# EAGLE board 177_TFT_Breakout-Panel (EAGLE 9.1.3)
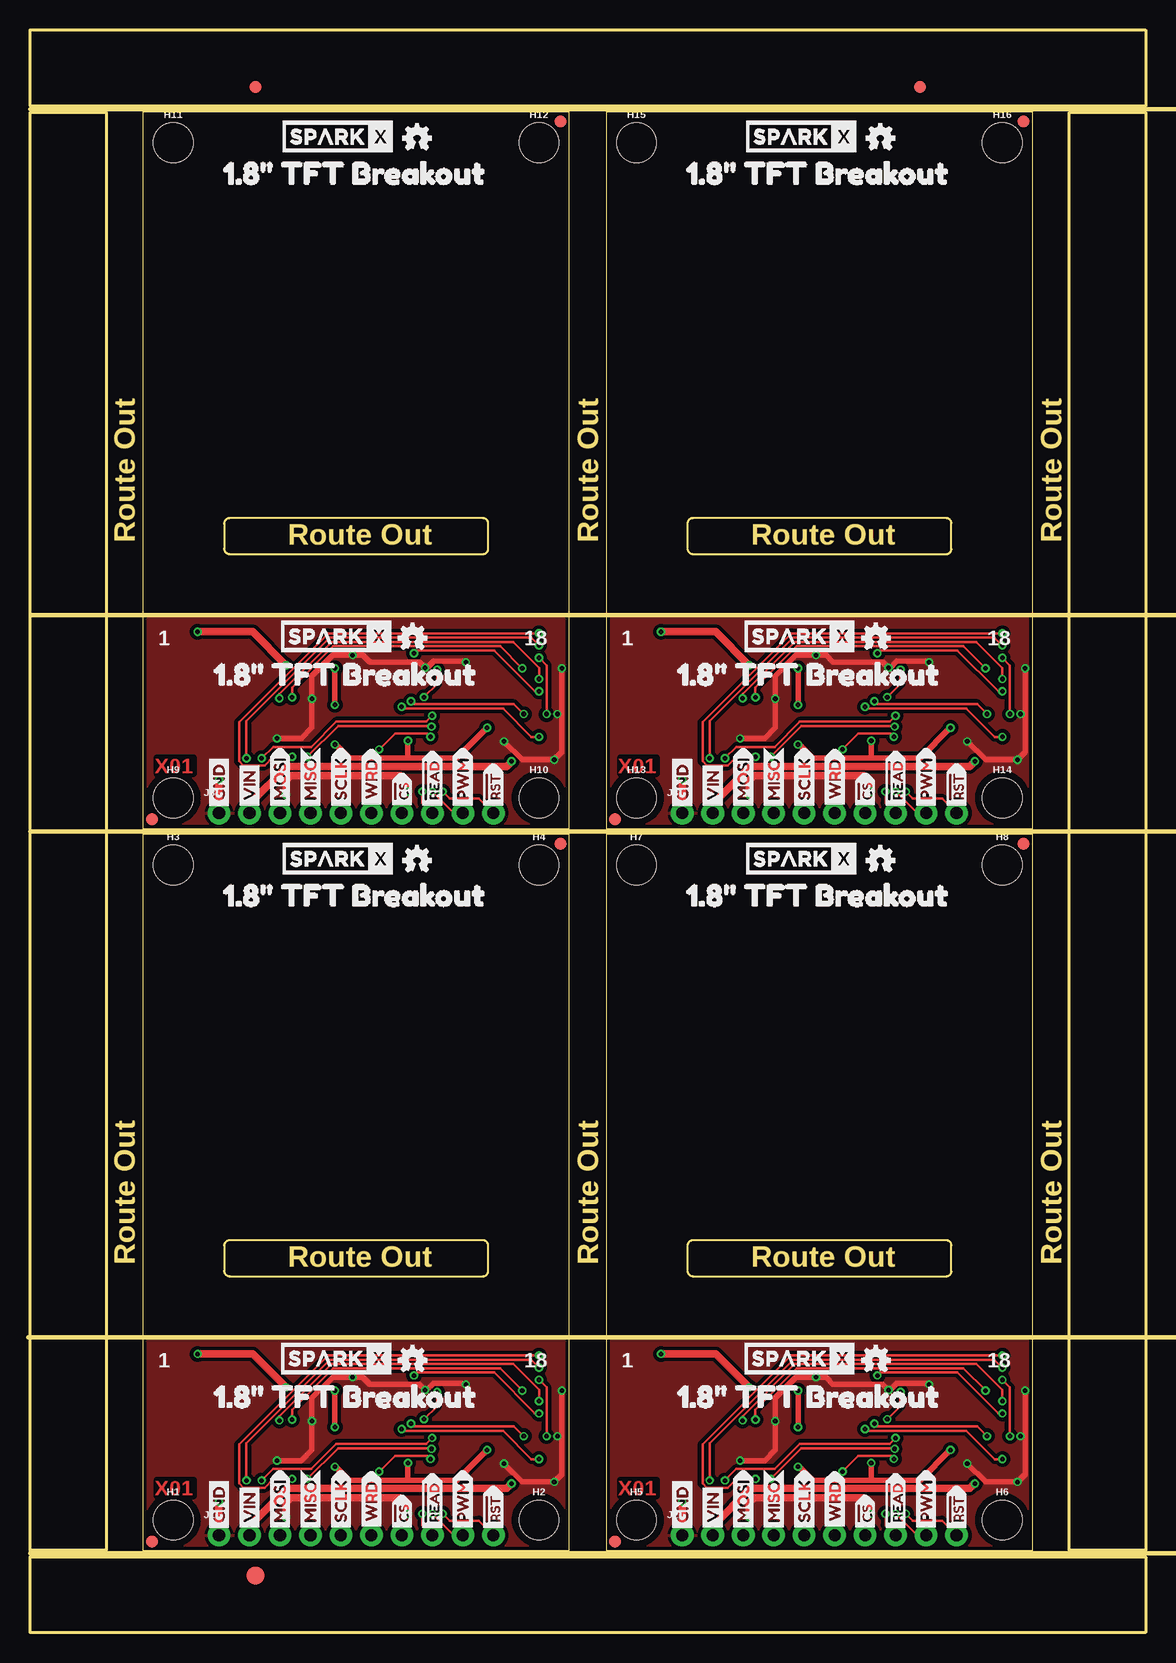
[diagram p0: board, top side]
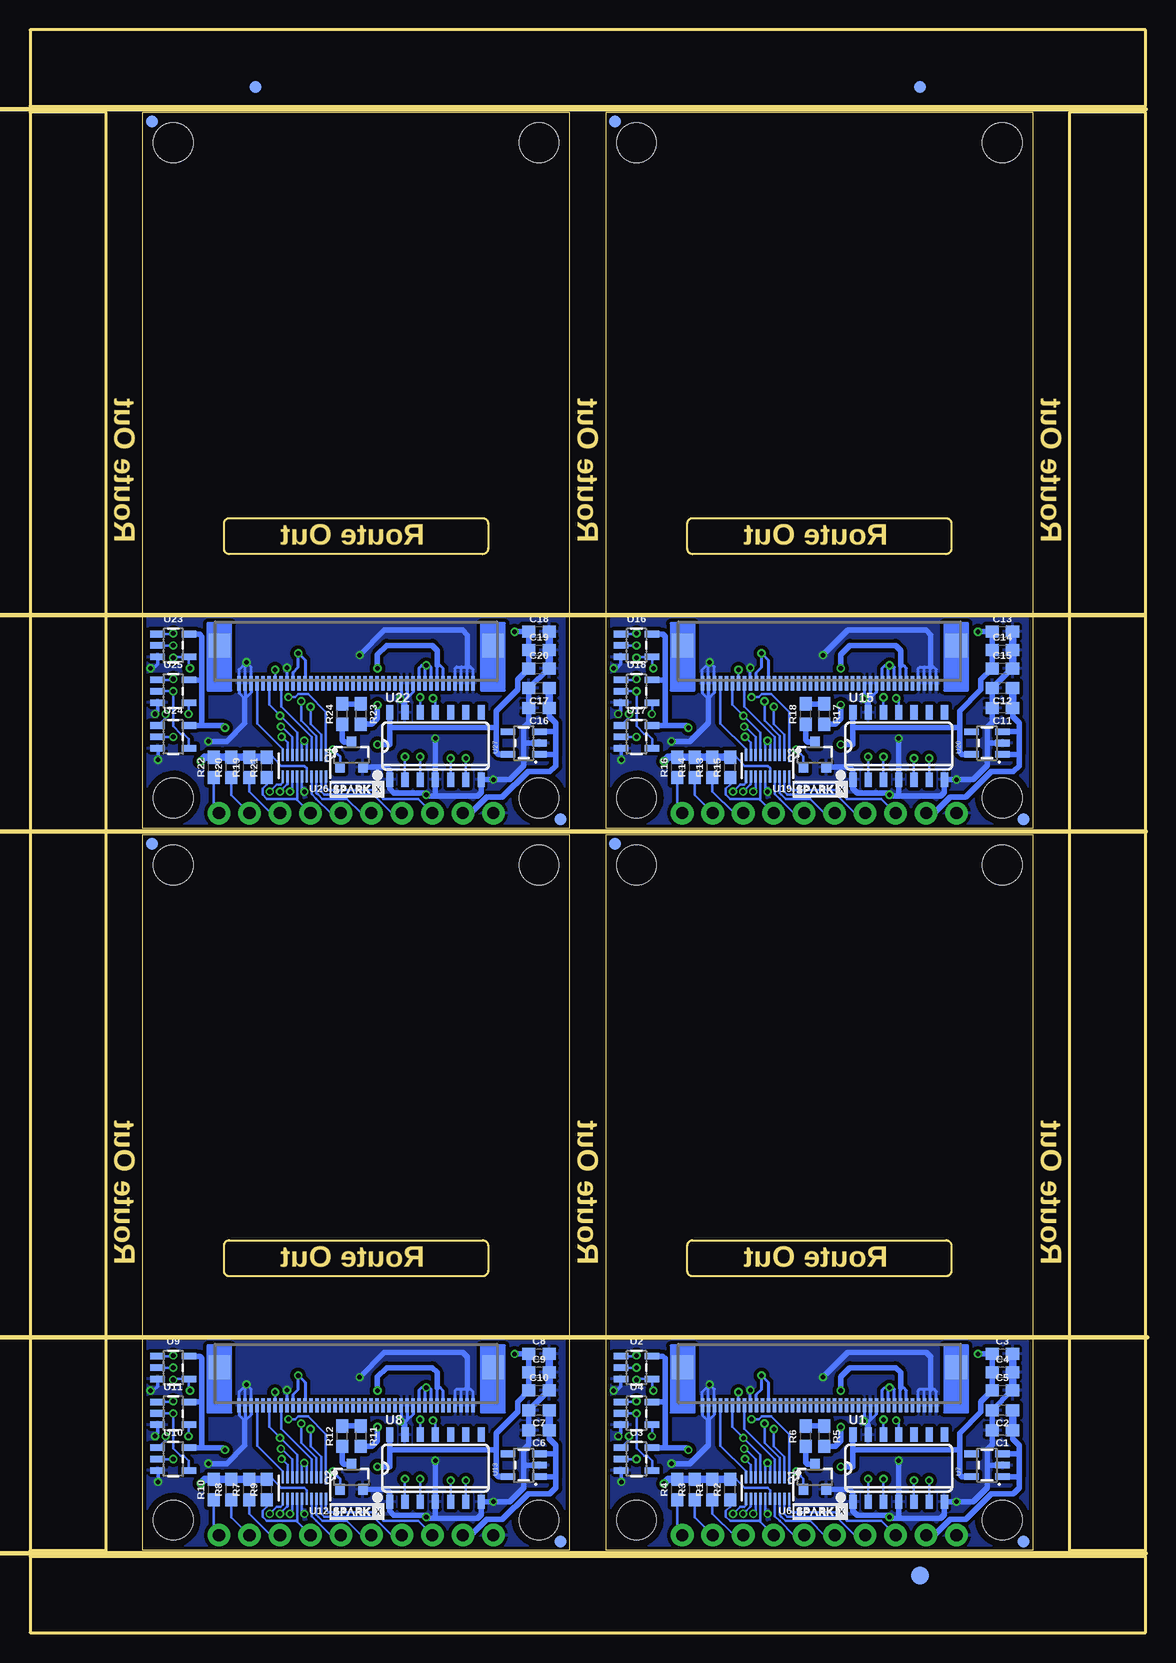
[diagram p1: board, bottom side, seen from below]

Size 92.96 x 133.6 mm. Coordinates in mm from the lower left corner, seen from the top.
Outline: 9.4,6.86 44.96,6.86 44.96,66.55 9.4,66.55 9.4,6.86
Outline: 48.01,6.86 83.57,6.86 83.57,66.55 48.01,66.55 48.01,6.86
Outline: 9.4,67.06 44.96,67.06 44.96,126.75 9.4,126.75 9.4,67.06
Outline: 48.01,67.06 83.57,67.06 83.57,126.75 48.01,126.75 48.01,67.06
Outline: 0,6.35 92.96,6.35 92.96,0 0,0 0,6.35
Outline: 86.61,126.75 92.96,126.75 92.96,6.86 86.61,6.86 86.61,126.75
Outline: 0,133.6 92.96,133.6 92.96,127.25 0,127.25 0,133.6
Outline: 0,126.75 6.35,126.75 6.35,6.86 0,6.86 0,126.75
Copper layers (1*16): Top 0.035mm / dielectric 1.5mm / Bottom 0.035mm
Design rules "SparkFun-2-layer-PCBWay-LIMIT": minimum track width 6mil, minimum drill 0.3mm, track to track 6mil, track to pad 6mil, pad to pad 6mil, via to via 6mil, smd to smd 6mil, copper to edge 6mil, drill to drill 6mil, minimum pad ring 6mil, minimum via ring 6mil, stop-mask expansion 4mil, vias tented up to drill 25mil, thermal gap 10mil
Milling: 37 lines

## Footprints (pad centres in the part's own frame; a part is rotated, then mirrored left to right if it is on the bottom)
0603 = smd 1.1 x 1: 1 -0.85,0; 2 0.85,0
FIDUCIAL-1X2 = smd 1 x 1: 1 0,0
FIDUCIAL-1.5X3 = smd 1.5 x 1.5: 1 0,0
STAND-OFF = hole 3.302: 0,0
1X10_NO_SILK = drill 1.016 pad 1.88: 1 0,0; 2 2.54,0; 3 5.08,0; 4 7.62,0; 5 10.16,0; 6 12.7,0; 7 15.24,0; 8 17.78,0; 9 20.32,0; 10 22.86,0
SOT23-3 = smd 0.8 x 0.9: 1 -0.95,-1; 2 0.95,-1; 3 0,1.1
SO14 = smd 0.6 x 1.2: 1 -3.175,-2.8; 2 -1.905,-2.8; 3 -0.635,-2.8; 4 0.635,-2.8; 5 1.905,-2.8; 6 3.175,-2.8; 7 4.445,-2.8; 8 4.445,2.8; 9 3.175,2.8; 10 1.905,2.8; 11 0.635,2.8; 12 -0.635,2.8; 13 -1.905,2.8; 14 -3.175,2.8
SOT23-5 = smd 0.55 x 1.2: 1 -0.95,-1.3; 2 0,-1.3; 3 0.95,-1.3; 4 0.95,1.3; 5 -0.95,1.3
FPC05040-17204 = smd 0.3 x 1.2: P$1 -9.75,0.6; P$2 -9.25,0.6; P$3 -8.75,0.6; P$4 -8.25,0.6; P$5 -7.75,0.6; P$6 -7.25,0.6; P$7 -6.75,0.6; P$8 -6.25,0.6; P$9 -5.75,0.6; P$10 -5.25,0.6; P$11 -4.75,0.6; P$12 -4.25,0.6; P$13 -3.75,0.6; P$14 -3.25,0.6; P$15 -2.75,0.6; P$16 -2.25,0.6; P$17 -1.75,0.6; P$18 -1.25,0.6; P$19 -0.75,0.6; P$20 -0.25,0.6; P$21 0.25,0.6; P$22 0.75,0.6; P$23 1.25,0.6; P$24 1.75,0.6; P$25 2.25,0.6; P$26 2.75,0.6; P$27 3.25,0.6; P$28 3.75,0.6; P$29 4.25,0.6; P$30 4.75,0.6; P$31 5.25,0.6; P$32 5.75,0.6; P$33 6.25,0.6; P$34 6.75,0.6; P$35 7.25,0.6; P$36 7.75,0.6; P$37 8.25,0.6; P$38 8.75,0.6; P$39 9.25,0.6; P$40 9.75,0.6 | smd 1.8 x 2: P$41 -11.4,-2.55; P$42 11.4,-2.55
UFDFN-20 = smd 0.2 x 1.1: 1 -1.8,-0.85 | smd 0.2 x 1: 2 -1.4,-0.9; 3 -1,-0.9; 4 -0.6,-0.9; 5 -0.2,-0.9; 6 0.2,-0.9; 7 0.6,-0.9; 8 1,-0.9; 9 1.4,-0.9; 10 1.8,-0.9; 11 1.8,0.9; 12 1.4,0.9; 13 1,0.9; 14 0.6,0.9; 15 0.2,0.9; 16 -0.2,0.9; 17 -0.6,0.9; 18 -1,0.9; 19 -1.4,0.9; 20 -1.8,0.9

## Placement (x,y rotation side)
C1  0.1uF  [0603]  11.94,16.89 180 bottom
C2  1.0uF  [0603]  11.94,18.54 180 bottom
C3  4.7uF  [0603]  11.94,23.24 0 bottom
C4  1.0uF  [0603]  11.94,21.72 0 bottom
C5  0.1uF  [0603]  11.94,20.19 0 bottom
C6  0.1uF  [0603]  50.55,16.89 180 bottom
C7  1.0uF  [0603]  50.55,18.54 180 bottom
C8  4.7uF  [0603]  50.55,23.24 0 bottom
C9  1.0uF  [0603]  50.55,21.72 0 bottom
C10  0.1uF  [0603]  50.55,20.19 0 bottom
C11  0.1uF  [0603]  11.94,77.09 180 bottom
C12  1.0uF  [0603]  11.94,78.74 180 bottom
C13  4.7uF  [0603]  11.94,83.44 0 bottom
C14  1.0uF  [0603]  11.94,81.92 0 bottom
C15  0.1uF  [0603]  11.94,80.39 0 bottom
C16  0.1uF  [0603]  50.55,77.09 180 bottom
C17  1.0uF  [0603]  50.55,78.74 180 bottom
C18  4.7uF  [0603]  50.55,83.44 0 bottom
C19  1.0uF  [0603]  50.55,81.92 0 bottom
C20  0.1uF  [0603]  50.55,80.39 0 bottom
E$1  [FIDUCIAL-1X2]  18.8,128.84 0 top
E$2  [FIDUCIAL-1X2]  18.8,128.84 0 bottom
E$3  [FIDUCIAL-1X2]  74.17,128.84 0 top
E$4  [FIDUCIAL-1X2]  74.17,128.84 0 bottom
E$5  [FIDUCIAL-1.5X3]  18.8,4.76 0 top
E$6  [FIDUCIAL-1.5X3]  18.8,4.76 0 bottom
FD1  FIDUCIAL1X2  [FIDUCIAL-1X2]  10.16,7.62 0 top
FD2  FIDUCIAL1X2  [FIDUCIAL-1X2]  44.2,65.79 0 top
FD3  FIDUCIAL1X2  [FIDUCIAL-1X2]  10.16,7.62 0 bottom
FD4  FIDUCIAL1X2  [FIDUCIAL-1X2]  44.2,65.79 0 bottom
FD5  FIDUCIAL1X2  [FIDUCIAL-1X2]  48.77,7.62 0 top
FD6  FIDUCIAL1X2  [FIDUCIAL-1X2]  82.8,65.79 0 top
FD7  FIDUCIAL1X2  [FIDUCIAL-1X2]  48.77,7.62 0 bottom
FD8  FIDUCIAL1X2  [FIDUCIAL-1X2]  82.8,65.79 0 bottom
FD9  FIDUCIAL1X2  [FIDUCIAL-1X2]  10.16,67.82 0 top
FD10  FIDUCIAL1X2  [FIDUCIAL-1X2]  44.2,125.98 0 top
FD11  FIDUCIAL1X2  [FIDUCIAL-1X2]  10.16,67.82 0 bottom
FD12  FIDUCIAL1X2  [FIDUCIAL-1X2]  44.2,125.98 0 bottom
FD13  FIDUCIAL1X2  [FIDUCIAL-1X2]  48.77,67.82 0 top
FD14  FIDUCIAL1X2  [FIDUCIAL-1X2]  82.8,125.98 0 top
FD15  FIDUCIAL1X2  [FIDUCIAL-1X2]  48.77,67.82 0 bottom
FD16  FIDUCIAL1X2  [FIDUCIAL-1X2]  82.8,125.98 0 bottom
H1  STAND-OFF  [STAND-OFF]  11.94,9.4 0 top
H2  STAND-OFF  [STAND-OFF]  42.42,9.4 0 top
H3  STAND-OFF  [STAND-OFF]  11.94,64.01 0 top
H4  STAND-OFF  [STAND-OFF]  42.42,64.01 0 top
H5  STAND-OFF  [STAND-OFF]  50.55,9.4 0 top
H6  STAND-OFF  [STAND-OFF]  81.03,9.4 0 top
H7  STAND-OFF  [STAND-OFF]  50.55,64.01 0 top
H8  STAND-OFF  [STAND-OFF]  81.03,64.01 0 top
H9  STAND-OFF  [STAND-OFF]  11.94,69.6 0 top
H10  STAND-OFF  [STAND-OFF]  42.42,69.6 0 top
H11  STAND-OFF  [STAND-OFF]  11.94,124.21 0 top
H12  STAND-OFF  [STAND-OFF]  42.42,124.21 0 top
H13  STAND-OFF  [STAND-OFF]  50.55,69.6 0 top
H14  STAND-OFF  [STAND-OFF]  81.03,69.6 0 top
H15  STAND-OFF  [STAND-OFF]  50.55,124.21 0 top
H16  STAND-OFF  [STAND-OFF]  81.03,124.21 0 top
J1  [1X10_NO_SILK]  15.75,8.13 0 top
J2  [1X10_NO_SILK]  54.36,8.13 0 top
J3  [1X10_NO_SILK]  15.75,68.33 0 top
J4  [1X10_NO_SILK]  54.36,68.33 0 top
LOGO1  OSHW-LOGOMINI  [OSHW-LOGO-MINI]  32.26,64.39 0 top
LOGO2  OSHW-LOGOMINI  [OSHW-LOGO-MINI]  31.88,22.73 0 top
LOGO3  OSHW-LOGOMINI  [OSHW-LOGO-MINI]  70.87,64.39 0 top
LOGO4  OSHW-LOGOMINI  [OSHW-LOGO-MINI]  70.48,22.73 0 top
LOGO5  OSHW-LOGOMINI  [OSHW-LOGO-MINI]  32.26,124.59 0 top
LOGO6  OSHW-LOGOMINI  [OSHW-LOGO-MINI]  31.88,82.93 0 top
LOGO7  OSHW-LOGOMINI  [OSHW-LOGO-MINI]  70.87,124.59 0 top
LOGO8  OSHW-LOGOMINI  [OSHW-LOGO-MINI]  70.48,82.93 0 top
Q1  220mA/50V/3.5Ω  [SOT23-3]  27.56,12.95 0 bottom
Q2  220mA/50V/3.5Ω  [SOT23-3]  66.17,12.95 0 bottom
Q3  220mA/50V/3.5Ω  [SOT23-3]  27.56,73.15 0 bottom
Q4  220mA/50V/3.5Ω  [SOT23-3]  66.17,73.15 0 bottom
R1  10k  [0603]  36.09,11.94 90 bottom
R2  10k  [0603]  34.62,11.94 90 bottom
R3  10k  [0603]  37.57,11.94 90 bottom
R4  10k  [0603]  39.04,11.94 90 bottom
R5  1  [0603]  26.8,16.38 270 bottom
R6  1  [0603]  28.32,16.38 90 bottom
R7  10k  [0603]  74.7,11.94 90 bottom
R8  10k  [0603]  76.17,11.94 90 bottom
R9  10k  [0603]  73.23,11.94 90 bottom
R10  10k  [0603]  77.65,11.94 90 bottom
R11  1  [0603]  65.41,16.38 270 bottom
R12  1  [0603]  66.93,16.38 90 bottom
R13  10k  [0603]  36.09,72.14 90 bottom
R14  10k  [0603]  37.57,72.14 90 bottom
R15  10k  [0603]  34.62,72.14 90 bottom
R16  10k  [0603]  39.04,72.14 90 bottom
R17  1  [0603]  26.8,76.58 270 bottom
R18  1  [0603]  28.32,76.58 90 bottom
R19  10k  [0603]  74.7,72.14 90 bottom
R20  10k  [0603]  76.17,72.14 90 bottom
R21  10k  [0603]  73.23,72.14 90 bottom
R22  10k  [0603]  77.65,72.14 90 bottom
R23  1  [0603]  65.41,76.58 270 bottom
R24  1  [0603]  66.93,76.58 90 bottom
U1  MC74AC125DG  [SO14]  21.21,13.72 0 bottom
U2  74LVC1G08SE  [SOT23-5]  42.42,22.1 270 bottom
U3  SN74AHC1G125  [SOT23-5]  42.42,14.48 270 bottom
U4  SN74AHC1G125  [SOT23-5]  42.42,18.29 270 bottom
U5  TF-LCM17723A-N  [FPC05040-17204]  27.18,19.56 180 bottom
U6  TXB0108DQSR  [UFDFN-20]  31.5,12.06 180 bottom
U7  3.3V  [SOT23-5]  13.21,13.97 90 bottom
U8  MC74AC125DG  [SO14]  59.82,13.72 0 bottom
U9  74LVC1G08SE  [SOT23-5]  81.03,22.1 270 bottom
U10  SN74AHC1G125  [SOT23-5]  81.03,14.48 270 bottom
U11  SN74AHC1G125  [SOT23-5]  81.03,18.29 270 bottom
U12  TXB0108DQSR  [UFDFN-20]  70.1,12.06 180 bottom
U13  3.3V  [SOT23-5]  51.82,13.97 90 bottom
U14  TF-LCM17723A-N  [FPC05040-17204]  65.79,19.56 180 bottom
U15  MC74AC125DG  [SO14]  21.21,73.91 0 bottom
U16  74LVC1G08SE  [SOT23-5]  42.42,82.3 270 bottom
U17  SN74AHC1G125  [SOT23-5]  42.42,74.68 270 bottom
U18  SN74AHC1G125  [SOT23-5]  42.42,78.49 270 bottom
U19  TXB0108DQSR  [UFDFN-20]  31.5,72.26 180 bottom
U20  3.3V  [SOT23-5]  13.21,74.17 90 bottom
U21  TF-LCM17723A-N  [FPC05040-17204]  27.18,79.76 180 bottom
U22  MC74AC125DG  [SO14]  59.82,73.91 0 bottom
U23  74LVC1G08SE  [SOT23-5]  81.03,82.3 270 bottom
U24  SN74AHC1G125  [SOT23-5]  81.03,74.68 270 bottom
U25  SN74AHC1G125  [SOT23-5]  81.03,78.49 270 bottom
U26  TXB0108DQSR  [UFDFN-20]  70.1,72.26 180 bottom
U27  3.3V  [SOT23-5]  51.82,74.17 90 bottom
U28  TF-LCM17723A-N  [FPC05040-17204]  65.79,79.76 180 bottom
U$1  [VIN2]  56.9,8.25 90 top
U$2  [GND1]  54.36,8.25 90 top
U$3  [VIN2]  18.29,8.25 90 top
U$4  [GND1]  15.75,8.25 90 top
U$5  [MOSI8]  20.83,8.25 90 top
U$6  [MISO9]  23.37,8.25 90 top
U$7  [PWM8]  36.07,8.25 90 top
U$8  [#READ7]  33.53,8.13 90 top
U$9  [#CS6]  30.99,8.13 90 top
U$10  [WRD9]  28.45,8.38 90 top
U$11  [SCLK7]  25.91,8.25 90 top
U$12  [#RST2]  38.61,8.13 90 top
U$13  [SPARKX-MEDIUM]  25.65,64.52 0 top
U$14  [1#8#_TFT_BREAKOUT10]  14.48,61.47 0 top
U$15  [1#8#_TFT_BREAKOUT10]  13.72,19.68 0 top
U$16  [PWM8]  74.68,8.25 90 top
U$17  [#READ7]  72.14,8.13 90 top
U$18  [#CS6]  69.6,8.13 90 top
U$19  [WRD9]  67.06,8.38 90 top
U$20  [MOSI8]  59.44,8.25 90 top
U$21  [MISO9]  61.98,8.25 90 top
U$22  [SCLK7]  64.52,8.25 90 top
U$23  [#RST2]  77.22,8.13 90 top
U$24  [SPARKX-MEDIUM]  64.14,22.86 0 top
U$25  [SPARKX-MEDIUM]  64.26,64.52 0 top
U$26  [1#8#_TFT_BREAKOUT10]  53.09,61.47 0 top
U$27  [1#8#_TFT_BREAKOUT10]  52.32,19.68 0 top
U$28  SPARKX-LOGO2  [SPARKX-TINY]  65.71,10.11 0 bottom
U$29  [VIN2]  18.29,68.45 90 top
U$30  [GND1]  15.75,68.45 90 top
U$31  [PWM8]  36.07,68.45 90 top
U$32  [#READ7]  33.53,68.33 90 top
U$33  [#CS6]  30.99,68.33 90 top
U$34  SPARKX-LOGO2  [SPARKX-TINY]  27.1,10.11 0 bottom
U$35  [WRD9]  28.45,68.58 90 top
U$36  [MOSI8]  20.83,68.45 90 top
U$37  [MISO9]  23.37,68.45 90 top
U$38  [SCLK7]  25.91,68.45 90 top
U$39  [#RST2]  38.61,68.33 90 top
U$40  [SPARKX-MEDIUM]  25.53,83.06 0 top
U$41  [SPARKX-MEDIUM]  25.65,124.71 0 top
U$42  [1#8#_TFT_BREAKOUT10]  14.48,121.67 0 top
U$43  [1#8#_TFT_BREAKOUT10]  13.72,79.88 0 top
U$44  SPARKX-LOGO2  [SPARKX-TINY]  27.1,70.31 0 bottom
U$45  [VIN2]  56.9,68.45 90 top
U$46  [GND1]  54.36,68.45 90 top
U$47  [PWM8]  74.68,68.45 90 top
U$48  [#READ7]  72.14,68.33 90 top
U$49  [#CS6]  69.6,68.33 90 top
U$50  [WRD9]  67.06,68.58 90 top
U$51  [SPARKX-MEDIUM]  25.53,22.86 0 top
U$52  [MOSI8]  59.44,68.45 90 top
U$53  [MISO9]  61.98,68.45 90 top
U$54  [SCLK7]  64.52,68.45 90 top
U$55  [#RST2]  77.22,68.33 90 top
U$56  [SPARKX-MEDIUM]  64.14,83.06 0 top
U$57  [SPARKX-MEDIUM]  64.26,124.71 0 top
U$58  [1#8#_TFT_BREAKOUT10]  53.09,121.67 0 top
U$59  [1#8#_TFT_BREAKOUT10]  52.32,79.88 0 top
U$60  SPARKX-LOGO2  [SPARKX-TINY]  65.71,70.31 0 bottom

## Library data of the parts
C1 C5 C6 C10 C11 C15 C16 C20 = SparkFun-Capacitors; PROD_ID: CAP-08390
C2 C4 C7 C9 C12 C14 C17 C19 = SparkFun-Capacitors; PROD_ID: CAP-00868
C3 C8 C13 C18 = SparkFun-Capacitors; PROD_ID: CAP-08280
E$1-E$4 FD1-FD16 LOGO1-LOGO8 = SparkFun-Aesthetics
E$5 E$6 = SparkFun-Retired
H1-H16 = SparkFun-Hardware
J1-J4 = SparkFun-Connectors; PROD_ID: CONN-11563
Q1-Q4 = SparkFun-DiscreteSemi; PROD_ID: TRANS-00830
R1-R4 R7-R10 R13-R16 R19-R22 = SparkFun-Resistors; PROD_ID: RES-00824
R5 R6 R11 R12 R17 R18 R23 R24 = SparkFun-Resistors; PROD_ID: RES-08269
U1 U8 U15 U22 = SparkFun-IC-Logic; PROD_ID: IC-08880
U2 U9 U16 U23 = SparkFun-IC-Logic; PROD_ID: IC-10841
U3 U4 U10 U11 U17 U18 U24 U25 = SparkFun-IC-Logic; PROD_ID: IC-11920
U5 U14 U21 U28 = all_displays
U6 U12 U19 U26 = SparkFun-IC-Comms; PROD_ID: IC-12292
U7 U13 U20 U27 = SparkFun-IC-Power; PROD_ID: VREG-12457
U$1-U$12 U$14-U$23 U$26 U$27 U$29-U$33 U$35-U$39 U$42 U$43 U$45-U$50 U$52-U$55 U$58 U$59 = buzzard_labels
U$13 U$24 U$25 U$28 U$34 U$40 U$41 U$44 U$51 U$56 U$57 U$60 = SparkX

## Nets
3.3V: C3.1 C4.1 C5.1 U1.14 U2.5 U3.5 U4.5 U5.P$8 U5.P$9 U5.P$10 U6.5 U6.6 U7.5
3.3V1: C8.1 C9.1 C10.1 U8.14 U9.5 U10.5 U11.5 U12.5 U12.6 U13.5 U14.P$8 U14.P$9 U14.P$10
3.3V2: C13.1 C14.1 C15.1 U15.14 U16.5 U17.5 U18.5 U19.5 U19.6 U20.5 U21.P$8 U21.P$9 U21.P$10
3.3V3: C18.1 C19.1 C20.1 U22.14 U23.5 U24.5 U25.5 U26.5 U26.6 U27.5 U28.P$8 U28.P$9 U28.P$10
!CS: U1.5 U5.P$35 U6.7
!CS1: U8.5 U12.7 U14.P$35
!CS2: U15.5 U19.7 U21.P$35
!CS3: U22.5 U26.7 U28.P$35
!CS_IN: J1.7 R2.1 U6.14
!CS_IN1: J2.7 R9.1 U12.14
!CS_IN2: J3.7 R15.1 U19.14
!CS_IN3: J4.7 R21.1 U26.14
!READ: U1.2 U6.8
!READ1: U8.2 U12.8
!READ2: U15.2 U19.8
!READ3: U22.2 U26.8
!READ_IN: J1.8 R1.1 U6.13
!READ_IN1: J2.8 R7.1 U12.13
!READ_IN2: J3.8 R13.1 U19.13
!READ_IN3: J4.8 R19.1 U26.13
!RESET: U5.P$37 U6.10
!RESET1: U12.10 U14.P$37
!RESET2: U19.10 U21.P$37
!RESET3: U26.10 U28.P$37
!RESET_IN: J1.10 R4.1 U6.11
!RESET_IN1: J2.10 R10.1 U12.11
!RESET_IN2: J3.10 R16.1 U19.11
!RESET_IN3: J4.10 R22.1 U26.11
DATA: U3.4 U4.2 U5.P$29 U5.P$31
DATA1: U10.4 U11.2 U14.P$29 U14.P$31
DATA2: U17.4 U18.2 U21.P$29 U21.P$31
DATA3: U24.4 U25.2 U28.P$29 U28.P$31
GND: C1.2 C2.2 C3.2 C4.2 C5.2 J1.1 Q1.2 U1.1 U1.4 U1.7 U1.13 U2.3 U3.3 U4.3 U5.P$1 U5.P$2 U5.P$3 U5.P$4 U5.P$11 U5.P$12 U5.P$13 U5.P$32 U5.P$38 U5.P$39 U5.P$40 U6.15 U7.2
GND1: C6.2 C7.2 C8.2 C9.2 C10.2 J2.1 Q2.2 U8.1 U8.4 U8.7 U8.13 U9.3 U10.3 U11.3 U12.15 U13.2 U14.P$1 U14.P$2 U14.P$3 U14.P$4 U14.P$11 U14.P$12 U14.P$13 U14.P$32 U14.P$38 U14.P$39 U14.P$40
GND2: C11.2 C12.2 C13.2 C14.2 C15.2 J3.1 Q3.2 U15.1 U15.4 U15.7 U15.13 U16.3 U17.3 U18.3 U19.15 U20.2 U21.P$1 U21.P$2 U21.P$3 U21.P$4 U21.P$11 U21.P$12 U21.P$13 U21.P$32 U21.P$38 U21.P$39 U21.P$40
GND3: C16.2 C17.2 C18.2 C19.2 C20.2 J4.1 Q4.2 U22.1 U22.4 U22.7 U22.13 U23.3 U24.3 U25.3 U26.15 U27.2 U28.P$1 U28.P$2 U28.P$3 U28.P$4 U28.P$11 U28.P$12 U28.P$13 U28.P$32 U28.P$38 U28.P$39 U28.P$40
LED_K: R5.2 U5.P$6 U5.P$7
LED_K1: R11.2 U14.P$6 U14.P$7
LED_K2: R17.2 U21.P$6 U21.P$7
LED_K3: R23.2 U28.P$6 U28.P$7
LED_PWM: Q1.1 U6.9
LED_PWM1: Q2.1 U12.9
LED_PWM2: Q3.1 U19.9
LED_PWM3: Q4.1 U26.9
LED_PWM_IN: J1.9 R3.1 U6.12
LED_PWM_IN1: J2.9 R8.1 U12.12
LED_PWM_IN2: J3.9 R14.1 U19.12
LED_PWM_IN3: J4.9 R20.1 U26.12
MISO: U4.4 U6.3
MISO1: U11.4 U12.3
MISO2: U18.4 U19.3
MISO3: U25.4 U26.3
MISO_IN: J1.5 U6.18
MISO_IN1: J2.5 U12.18
MISO_IN2: J3.5 U19.18
MISO_IN3: J4.5 U26.18
MOSI: U3.2 U6.2
MOSI1: U10.2 U12.2
MOSI2: U17.2 U19.2
MOSI3: U24.2 U26.2
MOSI_IN: J1.4 U6.19
MOSI_IN1: J2.4 U12.19
MOSI_IN2: J3.4 U19.19
MOSI_IN3: J4.4 U26.19
N$1: U1.6 U2.2
N$2: U1.3 U2.1
N$3: U1.12 U2.4 U3.1
N$4: R5.1 R6.2
N$5: Q1.3 R6.1
N$6: U8.6 U9.2
N$7: U8.3 U9.1
N$8: U1.11 U4.1
N$9: U8.12 U9.4 U10.1
N$10: U8.11 U11.1
N$11: R11.1 R12.2
N$12: Q2.3 R12.1
N$13: U15.6 U16.2
N$14: U15.3 U16.1
N$15: U15.12 U16.4 U17.1
N$16: U15.11 U18.1
N$17: R17.1 R18.2
N$18: Q3.3 R18.1
N$19: U22.6 U23.2
N$20: U22.3 U23.1
N$21: U22.12 U23.4 U24.1
N$22: U22.11 U25.1
N$23: R23.1 R24.2
N$24: Q4.3 R24.1
SCLK: U5.P$34 U6.1
SCLK1: U12.1 U14.P$34
SCLK2: U19.1 U21.P$34
SCLK3: U26.1 U28.P$34
SCLK_IN: J1.3 U6.20
SCLK_IN1: J2.3 U12.20
SCLK_IN2: J3.3 U19.20
SCLK_IN3: J4.3 U26.20
VIN: C1.1 C2.1 J1.2 R1.2 R2.2 R3.2 R4.2 U6.16 U7.1 U7.3
VIN1: C6.1 C7.1 J2.2 R7.2 R8.2 R9.2 R10.2 U12.16 U13.1 U13.3
VIN2: C11.1 C12.1 J3.2 R13.2 R14.2 R15.2 R16.2 U19.16 U20.1 U20.3
VIN3: C16.1 C17.1 J4.2 R19.2 R20.2 R21.2 R22.2 U26.16 U27.1 U27.3
WRD: U5.P$33 U6.4
WRD1: U12.4 U14.P$33
WRD2: U19.4 U21.P$33
WRD3: U26.4 U28.P$33
WRD_IN: J1.6 U6.17
WRD_IN1: J2.6 U12.17
WRD_IN2: J3.6 U19.17
WRD_IN3: J4.6 U26.17

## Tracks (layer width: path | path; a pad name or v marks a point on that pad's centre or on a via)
3.3V  (via drill 0.38)
  Top 0.457: v25.4,13.84 25.44,13.89 26.62,12.71 31.5,12.71 | v38.1,15.24 35.57,12.71 31.5,12.71 | v31.5,14.16 31.5,12.72 31.5,12.71
  Top 0.61: v13.97,23.24 18.54,23.24 v21.34,20.45
  Bottom 0.203: U6.5 31.3,13.96 v31.5,14.16 31.7,13.97 U6.6
  Bottom 0.254: U5.P$10 21.93,20.24 21.72,20.45 v21.34,20.45 | U5.P$9 21.43,20.36 v21.34,20.45 | v21.34,20.45 21.08,20.45 20.93,20.29 U5.P$8
  Bottom 0.457: v13.97,23.24 C3.1 C4.1 C5.1 13.72,19.26 13.72,18.41 15.49,16.64 15.49,15.24 | v38.1,15.24 38.29,15.43 40,15.43 | 40,15.43 U3.5 | U2.5 40.22,23.05 40.03,22.86 40.03,19.18 | 40.03,19.18 40.03,15.46 40,15.43 | U4.5 40.1,19.24 40.03,19.18 | 15.49,15.24 15.49,13.21 15.31,13.02 U7.5 | U1.14 24.38,15.24 | 24.38,15.24 24.38,13.84 v25.4,13.84 | 24.38,15.24 15.49,15.24
3.3V1  (via drill 0.38)
  Top 0.457: v64.01,13.84 64.05,13.89 65.22,12.71 70.1,12.71 | v76.71,15.24 74.18,12.71 70.1,12.71 | v70.11,14.16 70.11,12.72 70.1,12.71
  Top 0.61: v52.58,23.24 57.15,23.24 v59.94,20.45
  Bottom 0.203: U12.5 69.9,13.96 v70.11,14.16 70.3,13.97 U12.6
  Bottom 0.254: U14.P$10 60.54,20.24 60.33,20.45 v59.94,20.45 | U14.P$9 60.04,20.36 v59.94,20.45 | v59.94,20.45 59.69,20.45 59.54,20.29 U14.P$8
  Bottom 0.457: v52.58,23.24 C8.1 C9.1 C10.1 52.33,19.26 52.33,18.41 54.1,16.64 54.1,15.24 | v76.71,15.24 76.9,15.43 78.61,15.43 | 78.61,15.43 U10.5 | U9.5 78.83,23.05 78.64,22.86 78.64,19.18 | 78.64,19.18 78.64,15.46 78.61,15.43 | U11.5 78.7,19.24 78.64,19.18 | 54.1,15.24 54.1,13.21 53.91,13.02 U13.5 | U8.14 62.99,15.24 | 62.99,15.24 62.99,13.84 v64.01,13.84 | 62.99,15.24 54.1,15.24
3.3V2  (via drill 0.38)
  Top 0.457: v25.4,74.04 25.44,74.08 26.62,72.91 31.5,72.91 | v38.1,75.44 35.57,72.91 31.5,72.91 | v31.5,74.36 31.5,72.91
  Top 0.61: v13.97,83.44 18.54,83.44 v21.34,80.65
  Bottom 0.203: U19.5 31.3,74.16 v31.5,74.36 31.7,74.16 U19.6
  Bottom 0.254: U21.P$10 21.93,80.43 21.72,80.65 v21.34,80.65 | U21.P$9 21.43,80.55 v21.34,80.65 | v21.34,80.65 21.08,80.65 20.93,80.49 U21.P$8
  Bottom 0.457: v13.97,83.44 C13.1 C14.1 C15.1 13.72,79.46 13.72,78.61 15.49,76.84 15.49,75.44 | v38.1,75.44 38.29,75.63 40,75.63 | 40,75.63 U17.5 | U16.5 40.22,83.25 40.03,83.06 40.03,79.38 | 40.03,79.38 40.03,75.66 40,75.63 | U18.5 40.1,79.44 40.03,79.38 | 15.49,75.44 15.49,73.41 15.31,73.22 U20.5 | U15.14 24.38,75.44 | 24.38,75.44 24.38,74.04 v25.4,74.04 | 24.38,75.44 15.49,75.44
3.3V3  (via drill 0.38)
  Top 0.457: v64.01,74.04 64.05,74.08 65.22,72.91 70.1,72.91 | v76.71,75.44 74.18,72.91 70.1,72.91 | v70.11,74.36 70.11,72.91 70.1,72.91
  Top 0.61: v52.58,83.44 57.15,83.44 v59.94,80.65
  Bottom 0.203: U26.5 69.9,74.16 v70.11,74.36 70.3,74.16 U26.6
  Bottom 0.254: U28.P$10 60.54,80.43 60.33,80.65 v59.94,80.65 | U28.P$9 60.04,80.55 v59.94,80.65 | v59.94,80.65 59.69,80.65 59.54,80.49 U28.P$8
  Bottom 0.457: v52.58,83.44 C18.1 C19.1 C20.1 52.33,79.46 52.33,78.61 54.1,76.84 54.1,75.44 | v76.71,75.44 76.9,75.63 78.61,75.63 | 78.61,75.63 U24.5 | U23.5 78.83,83.25 78.64,83.06 78.64,79.38 | 78.64,79.38 78.64,75.66 78.61,75.63 | U25.5 78.7,79.44 78.64,79.38 | 54.1,75.44 54.1,73.41 53.91,73.22 U27.5 | U22.14 62.99,75.44 | 62.99,75.44 62.99,74.04 v64.01,74.04 | 62.99,75.44 54.1,75.44
!CS  (via drill 0.38)
  Top 0.203: v19.3,12.7 20.25,13.65 23.43,13.65 25.53,15.75 33.02,15.75 v33.52,16.25
  Bottom 0.203: v19.3,12.7 U1.5 | U5.P$35 34.43,17.16 v33.52,16.25 32.1,14.82 U6.7
!CS1  (via drill 0.38)
  Top 0.203: v57.91,12.7 58.86,13.65 62.04,13.65 64.14,15.75 71.63,15.75 v72.13,16.25
  Bottom 0.203: v57.91,12.7 U8.5 | U14.P$35 73.04,17.16 v72.13,16.25 70.7,14.82 U12.7
!CS2  (via drill 0.38)
  Top 0.203: v19.3,72.9 20.25,73.85 23.43,73.85 25.53,75.95 33.02,75.95 v33.52,76.44
  Bottom 0.203: v19.3,72.9 U15.5 | U21.P$35 34.43,77.35 v33.52,76.44 32.1,75.02 U19.7
!CS3  (via drill 0.38)
  Top 0.203: v57.91,72.9 58.86,73.85 62.04,73.85 64.14,75.95 71.63,75.95 v72.13,76.44
  Bottom 0.203: v57.91,72.9 U22.5 | U28.P$35 73.04,77.35 v72.13,76.44 70.7,75.02 U26.7
!CS_IN
  Bottom 0.203: U6.14 32.1,9.4 | 32.1,9.4 32.1,9.24 J1.7 | 32.1,9.4 32.17,9.32 34.62,9.32 34.97,9.67 34.97,10.17 34.62,10.52 R2.1
!CS_IN1
  Bottom 0.203: U12.14 70.7,9.4 | 70.7,9.4 70.7,9.24 J2.7 | 70.7,9.4 70.78,9.32 73.23,9.32 73.58,9.67 73.58,10.17 73.23,10.52 R9.1
!CS_IN2
  Bottom 0.203: U19.14 32.1,69.6 | 32.1,69.6 32.1,69.43 J3.7 | 32.1,69.6 32.17,69.52 34.62,69.52 34.97,69.87 34.97,70.36 34.62,70.72 R15.1
!CS_IN3
  Bottom 0.203: U26.14 70.7,69.6 | 70.7,69.6 70.7,69.43 J4.7 | 70.7,69.6 70.78,69.52 73.23,69.52 73.58,69.87 73.58,70.36 73.23,70.72 R21.1
!READ  (via drill 0.38)
  Top 0.203: v23.11,12.83 25.68,15.39 33.39,15.39 v33.45,15.33
  Bottom 0.203: v23.11,12.83 U1.2 | U6.8 32.5,14.45 33.38,15.33 v33.45,15.33
!READ1  (via drill 0.38)
  Top 0.203: v61.72,12.83 64.29,15.39 72,15.39 v72.06,15.33
  Bottom 0.203: v61.72,12.83 U8.2 | U12.8 71.1,14.45 71.98,15.33 v72.06,15.33
!READ2  (via drill 0.38)
  Top 0.203: v23.11,73.03 25.68,75.59 33.39,75.59 v33.45,75.53
  Bottom 0.203: v23.11,73.03 U15.2 | U19.8 32.5,74.65 33.38,75.53 v33.45,75.53
!READ3  (via drill 0.38)
  Top 0.203: v61.72,73.03 64.29,75.59 72,75.59 v72.06,75.53
  Bottom 0.203: v61.72,73.03 U22.2 | U26.8 71.1,74.65 71.98,75.53 v72.06,75.53
!READ_IN  (via drill 0.38)
  Top 0.203: v32.69,9.92 32.69,8.96 J1.8
  Bottom 0.203: R1.1 36.09,9.93 34.29,8.13 J1.8 | U6.13 32.5,10.12 v32.69,9.92
!READ_IN1  (via drill 0.38)
  Top 0.203: v71.3,9.92 71.3,8.96 J2.8
  Bottom 0.203: R7.1 74.7,9.93 72.9,8.13 J2.8 | U12.13 71.1,10.12 v71.3,9.92
!READ_IN2  (via drill 0.38)
  Top 0.203: v32.69,70.12 32.69,69.16 J3.8
  Bottom 0.203: R13.1 36.09,70.13 34.29,68.33 J3.8 | U19.13 32.5,70.31 v32.69,70.12
!READ_IN3  (via drill 0.38)
  Top 0.203: v71.3,70.12 71.3,69.16 J4.8
  Bottom 0.203: R19.1 74.7,70.13 72.9,68.33 J4.8 | U26.13 71.1,70.31 v71.3,70.12
!RESET
  Bottom 0.203: U6.10 33.3,13.46 35.43,15.59 U5.P$37
!RESET1
  Bottom 0.203: U12.10 71.9,13.46 74.04,15.59 U14.P$37
!RESET2
  Bottom 0.203: U19.10 33.3,73.66 35.43,75.79 U21.P$37
!RESET3
  Bottom 0.203: U26.10 71.9,73.66 74.04,75.79 U28.P$37
!RESET_IN  (via drill 0.38)
  Top 0.203: J1.10 37.4,9.33 34.96,9.33 v34.38,9.92
  Bottom 0.203: J1.10 39.04,8.56 R4.1 | U6.11 33.3,10.66 33.44,10.52 33.78,10.52 v34.38,9.92
!RESET_IN1  (via drill 0.38)
  Top 0.203: J2.10 76.01,9.33 73.57,9.33 v72.98,9.92
  Bottom 0.203: J2.10 77.65,8.56 R10.1 | U12.11 71.9,10.66 72.05,10.52 72.39,10.52 v72.98,9.92
!RESET_IN2  (via drill 0.38)
  Top 0.203: J3.10 37.4,69.53 34.96,69.53 v34.38,70.12
  Bottom 0.203: J3.10 39.04,68.76 R16.1 | U19.11 33.3,70.86 33.44,70.71 33.78,70.71 v34.38,70.12
!RESET_IN3  (via drill 0.38)
  Top 0.203: J4.10 76.01,69.53 73.57,69.53 v72.98,70.12
  Bottom 0.203: J4.10 77.65,68.76 R22.1 | U26.11 71.9,70.86 72.05,70.71 72.39,70.71 v72.98,70.12
DATA  (via drill 0.38)
  Top 0.203: v42.42,18.29 42.08,18.29 38.68,21.69 32.25,21.69 v32,21.45
  Bottom 0.203: U4.2 v42.42,18.29 42.42,15.37 41.78,14.73 41.53,14.73 41.12,14.32 U3.4
  Bottom 0.254: U5.P$29 31.43,20.87 v32,21.45 32,20.28 32.43,19.86 U5.P$31
DATA1  (via drill 0.38)
  Top 0.203: v81.03,18.29 80.69,18.29 77.29,21.69 70.85,21.69 v70.61,21.45
  Bottom 0.203: U11.2 v81.03,18.29 81.03,15.37 80.39,14.73 80.14,14.73 79.73,14.32 U10.4
  Bottom 0.254: U14.P$29 70.04,20.87 v70.61,21.45 70.61,20.28 71.04,19.86 U14.P$31
DATA2  (via drill 0.38)
  Top 0.203: v42.42,78.49 42.08,78.49 38.68,81.89 32.25,81.89 v32,81.65
  Bottom 0.203: U18.2 v42.42,78.49 42.42,75.56 41.78,74.93 41.53,74.93 41.12,74.52 U17.4
  Bottom 0.254: U21.P$29 31.43,81.07 v32,81.65 32,80.48 32.43,80.06 U21.P$31
DATA3  (via drill 0.38)
  Top 0.203: v81.03,78.49 80.69,78.49 77.29,81.89 70.85,81.89 v70.61,81.65
  Bottom 0.203: U25.2 v81.03,78.49 81.03,75.56 80.39,74.93 80.14,74.93 79.73,74.52 U24.4
  Bottom 0.254: U28.P$29 70.04,81.07 v70.61,81.65 70.61,80.48 71.04,80.06 U28.P$31
GND  (via drill 0.38)
  Top 0.457: 44.32,16.38 44.32,13.21 v43.69,12.57 41.02,12.57 v39.5,14.1 | 44.32,16.38 v44.32,20.19 | v43.94,16.38 44.32,16.38 | v36.32,20.7 36.23,20.79 33.63,20.79 33.07,20.23 v32.93,20.23 32.44,20.73 28.3,20.73 27.73,21.3 v26.89,21.3 25.22,21.3 23.49,19.57 v23.49,17.65 23.49,15.24 22.61,14.35 v20.57,14.35
  Top 0.61: J1.1 v15.75,10.92 | v21.34,9.65 21.34,10.86 21.74,11.27 30.86,11.27 31.5,10.63 v31.5,9.91
  Bottom 0.203: U6.15 31.7,10.11 v31.5,9.91 | 23.43,17.72 v23.49,17.65 | v32.93,20.23
  Bottom 0.254: 18.41,20.32 18.8,20.32 18.93,20.19 U5.P$4 | 18.41,20.32 17.91,20.32 | 17.91,20.32 17.65,20.32 17.43,20.09 U5.P$1 | 17.91,20.32 17.93,20.3 U5.P$2 | 23.43,17.72 v23.49,17.65 | U5.P$13 23.43,17.72 | 23.43,17.72 v23.49,17.65 | U5.P$11 22.43,18.21 22.99,17.65 | 22.99,17.65 v23.49,17.65 | U5.P$12 22.93,17.71 22.99,17.65 | U5.P$32 v32.93,20.23 | v36.32,20.7 36.93,20.09 U5.P$40 36.93,18.13 36.45,17.65 | v36.32,20.7 35.93,20.31 U5.P$38 35.93,18.17 36.45,17.65 | v36.32,20.7 36.43,20.59 U5.P$39 36.43,17.67 36.45,17.65 | U5.P$3 18.43,20.31 18.41,20.32
  Bottom 0.305: U2.3 43.72,20.54 44.07,20.19 v44.32,20.19 | U4.3 43.72,16.61 v43.94,16.38 | U3.3 43.69,13.5 v43.69,12.57
  Bottom 0.457: C5.2 11.14,20.19 C2.2 C1.2 12.79,15.66 13.21,15.24 13.21,13.97 | U1.13 23.11,17.27 v23.49,17.65 | U7.2 13.21,13.97 | v39.5,14.1 37.97,14.1 36.45,15.62 36.45,17.65 | 20.57,9.56 17.05,9.56 16.76,9.84 U1.7 v15.75,10.92 14.38,10.92 13.21,12.09 13.21,13.97 | 20.57,9.56 21.24,9.56 v21.34,9.65 21.49,9.8 24.03,9.8 24.38,10.16 U1.1 24.38,11.68 24.65,11.95 Q1.2 | 20.57,9.56 U1.4 v20.57,14.35 | 17.91,20.32 17.91,22.99 18.29,23.37 24.82,23.37 v26.89,21.3
  Bottom 0.61: C3.2 C4.2 C5.2
  pour Bottom (isolate 0.305): 44.96,6.86 44.96,24.64 9.4,24.64 9.4,6.86
  pour Top (isolate 0.305): 44.96,6.86 44.96,24.64 9.4,24.64 9.4,6.86
GND1  (via drill 0.38)
  Top 0.457: 82.93,16.38 82.93,13.21 v82.3,12.57 79.63,12.57 v78.1,14.1 | 82.93,16.38 v82.93,20.19 | v82.55,16.38 82.93,16.38 | v74.93,20.7 74.84,20.79 72.24,20.79 71.68,20.23 v71.54,20.23 71.05,20.73 66.91,20.73 66.34,21.3 v65.49,21.3 63.83,21.3 62.1,19.57 v62.1,17.65 62.1,15.24 61.21,14.35 v59.18,14.35
  Top 0.61: J2.1 v54.36,10.92 | v59.94,9.65 59.94,10.86 60.35,11.27 69.47,11.27 70.1,10.63 v70.1,9.91
  Bottom 0.203: U12.15 70.3,10.11 v70.1,9.91 | 62.04,17.72 v62.1,17.65 | v71.54,20.23
  Bottom 0.254: 57.02,20.32 57.4,20.32 57.54,20.19 U14.P$4 | 57.02,20.32 56.52,20.32 | 56.52,20.32 56.26,20.32 56.04,20.09 U14.P$1 | 56.52,20.32 56.54,20.3 U14.P$2 | 62.04,17.72 v62.1,17.65 | U14.P$13 62.04,17.72 | 62.04,17.72 v62.1,17.65 | U14.P$11 61.04,18.21 61.59,17.65 | 61.59,17.65 v62.1,17.65 | U14.P$12 61.54,17.71 61.59,17.65 | U14.P$32 v71.54,20.23 | v74.93,20.7 75.54,20.09 U14.P$40 75.54,18.13 75.06,17.65 | v74.93,20.7 74.54,20.31 U14.P$38 74.54,18.17 75.06,17.65 | v74.93,20.7 75.04,20.59 U14.P$39 75.04,17.67 75.06,17.65 | U14.P$3 57.04,20.31 57.02,20.32
  Bottom 0.305: U9.3 82.33,20.54 82.68,20.19 v82.93,20.19 | U11.3 82.33,16.61 v82.55,16.38 | U10.3 82.3,13.5 v82.3,12.57
  Bottom 0.457: C10.2 49.75,20.19 C7.2 C6.2 51.4,15.66 51.82,15.24 51.82,13.97 | U8.13 61.72,17.27 v62.1,17.65 | U13.2 51.82,13.97 | v78.1,14.1 76.58,14.1 75.06,15.62 75.06,17.65 | 59.18,9.56 55.66,9.56 55.37,9.84 U8.7 v54.36,10.92 52.98,10.92 51.82,12.09 51.82,13.97 | 59.18,9.56 59.85,9.56 v59.94,9.65 60.1,9.8 62.64,9.8 62.99,10.16 U8.1 62.99,11.68 63.26,11.95 Q2.2 | 59.18,9.56 U8.4 v59.18,14.35 | 56.52,20.32 56.52,22.99 56.9,23.37 63.42,23.37 v65.49,21.3
  Bottom 0.61: C8.2 C9.2 C10.2
  pour Bottom (isolate 0.305): 83.57,6.86 83.57,24.64 48.01,24.64 48.01,6.86
  pour Top (isolate 0.305): 83.57,6.86 83.57,24.64 48.01,24.64 48.01,6.86
GND2  (via drill 0.38)
  Top 0.457: 44.32,76.58 44.32,73.41 v43.69,72.77 41.02,72.77 v39.5,74.3 | 44.32,76.58 v44.32,80.39 | v43.94,76.58 44.32,76.58 | v36.32,80.9 36.23,80.99 33.63,80.99 33.07,80.43 v32.93,80.43 32.44,80.92 28.3,80.92 27.73,81.5 v26.89,81.5 25.22,81.5 23.49,79.77 v23.49,77.85 23.49,75.44 22.61,74.55 v20.57,74.55
  Top 0.61: J3.1 v15.75,71.12 | v21.34,69.85 21.34,71.06 21.74,71.46 30.86,71.46 31.5,70.83 v31.5,70.1
  Bottom 0.203: U19.15 31.7,70.3 v31.5,70.1 | 23.43,77.92 v23.49,77.85 | v32.93,80.43
  Bottom 0.254: 18.41,80.52 18.8,80.52 18.93,80.39 U21.P$4 | 18.41,80.52 17.91,80.52 | 17.91,80.52 17.65,80.52 17.43,80.29 U21.P$1 | 17.91,80.52 17.93,80.5 U21.P$2 | 23.43,77.92 v23.49,77.85 | U21.P$13 23.43,77.92 | 23.43,77.92 v23.49,77.85 | U21.P$11 22.43,78.41 22.99,77.85 | 22.99,77.85 v23.49,77.85 | U21.P$12 22.93,77.91 22.99,77.85 | U21.P$32 v32.93,80.43 | v36.32,80.9 36.93,80.29 U21.P$40 36.93,78.33 36.45,77.85 | v36.32,80.9 35.93,80.51 U21.P$38 35.93,78.37 36.45,77.85 | v36.32,80.9 36.43,80.79 U21.P$39 36.43,77.87 36.45,77.85 | U21.P$3 18.43,80.51 18.41,80.52
  Bottom 0.305: U16.3 43.72,80.74 44.07,80.39 v44.32,80.39 | U18.3 43.72,76.81 v43.94,76.58 | U17.3 43.69,73.7 v43.69,72.77
  Bottom 0.457: C15.2 11.14,80.39 C12.2 C11.2 12.79,75.86 13.21,75.44 13.21,74.17 | U15.13 23.11,77.47 v23.49,77.85 | U20.2 13.21,74.17 | v39.5,74.3 37.97,74.3 36.45,75.82 36.45,77.85 | 20.57,69.75 17.05,69.75 16.76,70.04 U15.7 v15.75,71.11 v15.75,71.12 14.38,71.12 13.21,72.29 13.21,74.17 | 20.57,69.75 21.24,69.75 v21.34,69.85 21.49,70 24.03,70 24.38,70.36 U15.1 24.38,71.88 24.65,72.15 Q3.2 | 20.57,69.75 U15.4 v20.57,74.55 | 17.91,80.52 17.91,83.19 18.29,83.57 24.82,83.57 v26.89,81.5
  Bottom 0.61: C13.2 C14.2 C15.2
  pour Bottom (isolate 0.305): 44.96,67.06 44.96,84.84 9.4,84.84 9.4,67.06
  pour Top (isolate 0.305): 44.96,67.06 44.96,84.84 9.4,84.84 9.4,67.06
GND3  (via drill 0.38)
  Top 0.457: 82.93,76.58 82.93,73.41 v82.3,72.77 79.63,72.77 v78.1,74.3 | 82.93,76.58 v82.93,80.39 | v82.55,76.58 82.93,76.58 | v74.93,80.9 74.84,80.99 72.24,80.99 71.68,80.43 v71.54,80.43 71.05,80.92 66.91,80.92 66.34,81.5 v65.49,81.5 63.83,81.5 62.1,79.77 v62.1,77.85 62.1,75.44 61.21,74.55 v59.18,74.55
  Top 0.61: J4.1 v54.36,71.12 | v59.94,69.85 59.94,71.06 60.35,71.46 69.47,71.46 70.1,70.83 v70.1,70.1
  Bottom 0.203: U26.15 70.3,70.3 v70.1,70.1 | 62.04,77.92 v62.1,77.85 | v71.54,80.43
  Bottom 0.254: 57.02,80.52 57.4,80.52 57.54,80.39 U28.P$4 | 57.02,80.52 56.52,80.52 | 56.52,80.52 56.26,80.52 56.04,80.29 U28.P$1 | 56.52,80.52 56.54,80.5 U28.P$2 | 62.04,77.92 v62.1,77.85 | U28.P$13 62.04,77.92 | 62.04,77.92 v62.1,77.85 | U28.P$11 61.04,78.41 61.59,77.85 | 61.59,77.85 v62.1,77.85 | U28.P$12 61.54,77.91 61.59,77.85 | U28.P$32 v71.54,80.43 | v74.93,80.9 75.54,80.29 U28.P$40 75.54,78.33 75.06,77.85 | v74.93,80.9 74.54,80.51 U28.P$38 74.54,78.37 75.06,77.85 | v74.93,80.9 75.04,80.79 U28.P$39 75.04,77.87 75.06,77.85 | U28.P$3 57.04,80.51 57.02,80.52
  Bottom 0.305: U23.3 82.33,80.74 82.68,80.39 v82.93,80.39 | U25.3 82.33,76.81 v82.55,76.58 | U24.3 82.3,73.7 v82.3,72.77
  Bottom 0.457: C20.2 49.75,80.39 C17.2 C16.2 51.4,75.86 51.82,75.44 51.82,74.17 | U22.13 61.72,77.47 v62.1,77.85 | U27.2 51.82,74.17 | v78.1,74.3 76.58,74.3 75.06,75.82 75.06,77.85 | 59.18,69.75 55.66,69.75 55.37,70.04 U22.7 v54.36,71.11 v54.36,71.12 52.98,71.12 51.82,72.29 51.82,74.17 | 59.18,69.75 59.85,69.75 v59.94,69.85 60.1,70 62.64,70 62.99,70.36 U22.1 62.99,71.88 63.26,72.15 Q4.2 | 59.18,69.75 U22.4 v59.18,74.55 | 56.52,80.52 56.52,83.19 56.9,83.57 63.42,83.57 v65.49,81.5
  Bottom 0.61: C18.2 C19.2 C20.2
  pour Bottom (isolate 0.305): 83.57,67.06 83.57,84.84 48.01,84.84 48.01,67.06
  pour Top (isolate 0.305): 83.57,67.06 83.57,84.84 48.01,84.84 48.01,67.06
LED_K  (via drill 0.38)
  Top 0.457: v25.4,17.14 v25.4,20.19
  Bottom 0.254: U5.P$7 20.43,20.42 20.42,20.42 20.16,20.42 19.93,20.18 U5.P$6
  Bottom 0.457: 20.42,20.42 20.42,21.69 20.83,22.1 24.64,22.1 25.4,21.34 v25.4,20.19 | R5.2 25.87,15.53 25.4,16 v25.4,17.14
LED_K1  (via drill 0.38)
  Top 0.457: v64.01,17.14 v64.01,20.19
  Bottom 0.254: U14.P$7 59.04,20.42 59.03,20.42 58.77,20.42 58.54,20.18 U14.P$6
  Bottom 0.457: 59.03,20.42 59.03,21.69 59.44,22.1 63.25,22.1 64.01,21.34 v64.01,20.19 | R11.2 64.48,15.53 64.01,16 v64.01,17.14
LED_K2  (via drill 0.38)
  Top 0.457: v25.4,77.34 v25.4,80.39
  Bottom 0.254: U21.P$7 20.43,80.62 20.42,80.62 20.16,80.62 19.93,80.38 U21.P$6
  Bottom 0.457: 20.42,80.62 20.42,81.89 20.83,82.3 24.64,82.3 25.4,81.53 v25.4,80.39 | R17.2 25.87,75.73 25.4,76.2 v25.4,77.34
LED_K3  (via drill 0.38)
  Top 0.457: v64.01,77.34 v64.01,80.39
  Bottom 0.254: U28.P$7 59.04,80.62 59.03,80.62 58.77,80.62 58.54,80.38 U28.P$6
  Bottom 0.457: 59.03,80.62 59.03,81.89 59.44,82.3 63.25,82.3 64.01,81.53 v64.01,80.39 | R23.2 64.48,75.73 64.01,76.2 v64.01,77.34
LED_PWM  (via drill 0.38)
  Top 0.203: v29.1,13.44 30.42,14.76 33.12,14.76 v33.38,14.49
  Bottom 0.203: Q1.1 28.51,12.83 28.73,13.05 28.73,13.07 v29.1,13.44 | U6.9 32.9,13.84 32.9,14.01 v33.38,14.49
LED_PWM1  (via drill 0.38)
  Top 0.203: v67.71,13.44 69.03,14.76 71.72,14.76 v71.99,14.49
  Bottom 0.203: Q2.1 67.12,12.83 67.34,13.05 67.34,13.07 v67.71,13.44 | U12.9 71.5,13.84 71.5,14.01 v71.99,14.49
LED_PWM2  (via drill 0.38)
  Top 0.203: v29.1,73.64 30.42,74.96 33.12,74.96 v33.38,74.69
  Bottom 0.203: Q3.1 28.51,73.03 28.73,73.25 28.73,73.27 v29.1,73.64 | U19.9 32.9,74.04 32.9,74.21 v33.38,74.69
LED_PWM3  (via drill 0.38)
  Top 0.203: v67.71,73.64 69.03,74.96 71.72,74.96 v71.99,74.69
  Bottom 0.203: Q4.1 67.12,73.03 67.34,73.25 67.34,73.27 v67.71,73.64 | U26.9 71.5,74.04 71.5,74.21 v71.99,74.69
LED_PWM_IN  (via drill 0.38)
  Top 0.203: v33.53,9.92 35.32,8.13 J1.9
  Bottom 0.203: J1.9 37.57,9.63 R3.1 | v33.53,9.92 33.29,10.16 33.29,10.17 32.94,10.52 32.93,10.52 32.9,10.55 U6.12
LED_PWM_IN1  (via drill 0.38)
  Top 0.203: v72.14,9.92 73.93,8.13 J2.9
  Bottom 0.203: J2.9 76.17,9.63 R8.1 | v72.14,9.92 71.9,10.16 71.9,10.17 71.55,10.52 71.54,10.52 71.5,10.55 U12.12
LED_PWM_IN2  (via drill 0.38)
  Top 0.203: v33.53,70.12 35.32,68.33 J3.9
  Bottom 0.203: J3.9 37.57,69.83 R14.1 | v33.53,70.12 33.29,70.36 32.94,70.71 32.93,70.71 32.9,70.75 U19.12
LED_PWM_IN3  (via drill 0.38)
  Top 0.203: v72.14,70.12 73.93,68.33 J4.9
  Bottom 0.203: J4.9 76.17,69.83 R20.1 | v72.14,70.12 71.9,70.36 71.55,70.71 71.54,70.71 71.5,70.75 U26.12
MISO  (via drill 0.38)
  Top 0.203: v41.15,16.38 40.33,17.2 31.99,17.2 v31.75,17.44
  Bottom 0.203: v41.15,16.38 41.12,16.41 U4.4 | U6.3 30.5,14.57 31.75,15.82 v31.75,17.44
MISO1  (via drill 0.38)
  Top 0.203: v79.76,16.38 78.94,17.2 70.6,17.2 v70.36,17.44
  Bottom 0.203: v79.76,16.38 79.73,16.41 U11.4 | U12.3 69.1,14.57 70.36,15.82 v70.36,17.44
MISO2  (via drill 0.38)
  Top 0.203: v41.15,76.58 40.33,77.4 31.99,77.4 v31.75,77.64
  Bottom 0.203: v41.15,76.58 41.12,76.61 U18.4 | U19.3 30.5,74.77 31.75,76.02 v31.75,77.64
MISO3  (via drill 0.38)
  Top 0.203: v79.76,76.58 78.94,77.4 70.6,77.4 v70.36,77.64
  Bottom 0.203: v79.76,76.58 79.73,76.61 U25.4 | U26.3 69.1,74.77 70.36,76.02 v70.36,77.64
MISO_IN
  Bottom 0.203: U6.18 30.5,9.82 30.35,9.68 29.99,9.32 27.95,9.32 26.76,8.13 J1.5
MISO_IN1
  Bottom 0.203: U12.18 69.1,9.82 68.96,9.68 68.95,9.68 68.6,9.32 66.56,9.32 65.37,8.13 J2.5
MISO_IN2
  Bottom 0.203: U19.18 30.5,70.02 30.35,69.88 29.99,69.52 27.95,69.52 26.76,68.33 J3.5
MISO_IN3
  Bottom 0.203: U26.18 69.1,70.02 68.96,69.88 68.95,69.88 68.6,69.52 66.56,69.52 65.37,68.33 J4.5
MOSI  (via drill 0.38)
  Top 0.203: v42.42,14.48 41.78,14.48 39.42,16.84 31.11,16.84 v30.97,16.98
  Bottom 0.203: v42.42,14.48 U3.2 | U6.2 30.1,14.67 30.97,15.55 v30.97,16.98
MOSI1  (via drill 0.38)
  Top 0.203: v81.03,14.48 80.39,14.48 78.03,16.84 69.72,16.84 v69.58,16.98
  Bottom 0.203: v81.03,14.48 U10.2 | U12.2 68.7,14.67 69.58,15.55 v69.58,16.98
MOSI2  (via drill 0.38)
  Top 0.203: v42.42,74.68 41.78,74.68 39.42,77.04 31.11,77.04 v30.97,77.18
  Bottom 0.203: v42.42,74.68 U17.2 | U19.2 30.1,74.87 30.97,75.75 v30.97,77.18
MOSI3  (via drill 0.38)
  Top 0.203: v81.03,74.68 80.39,74.68 78.03,77.04 69.72,77.04 v69.58,77.18
  Bottom 0.203: v81.03,74.68 U24.2 | U26.2 68.7,74.87 69.58,75.75 v69.58,77.18
MOSI_IN
  Bottom 0.203: U6.19 30.1,9.93 29.84,9.68 25.77,9.68 24.22,8.13 J1.4
MOSI_IN1
  Bottom 0.203: U12.19 68.7,9.93 68.45,9.68 64.38,9.68 62.83,8.13 J2.4
MOSI_IN2
  Bottom 0.203: U19.19 30.1,70.13 29.84,69.88 25.77,69.88 24.22,68.33 J3.4
MOSI_IN3
  Bottom 0.203: U26.19 68.7,70.13 68.45,69.88 64.38,69.88 62.83,68.33 J4.4
N$1  (via drill 0.38)
  Top 0.203: v42.42,22.1 41.76,22.76 24.99,22.76 18.03,15.8 v18.03,12.7
  Bottom 0.203: U2.2 v42.42,22.1 | v18.03,12.7 U1.6
N$2  (via drill 0.38)
  Top 0.203: v21.84,12.83 20.27,12.83 19.55,12.1 17.79,12.1 17.44,12.45 17.44,15.7 24.85,23.11 v42.42,23.11
  Bottom 0.203: U2.1 42.48,23.05 v42.42,23.11 | v21.84,12.83 U1.3
N$3  (via drill 0.38)
  Top 0.203: v41.02,20.19 39.17,22.05 25.29,22.05 21.84,18.6 v21.84,17.78 | v43.05,16.38 43.05,20.45 v42.42,21.08
  Bottom 0.203: v42.42,21.08 42.35,21.15 U2.4 41.12,20.29 v41.02,20.19 | v21.84,17.78 U1.12 | U3.1 43.05,16.09 v43.05,16.38
N$4
  Bottom 0.457: R6.2 R5.1
N$5
  Bottom 0.457: Q1.3 28.15,14.05 28.32,14.22 R6.1
N$6  (via drill 0.38)
  Top 0.203: v81.03,22.1 80.37,22.76 63.6,22.76 56.64,15.8 v56.64,12.7
  Bottom 0.203: U9.2 v81.03,22.1 | v56.64,12.7 U8.6
N$7  (via drill 0.38)
  Top 0.203: v60.45,12.83 58.88,12.83 58.16,12.1 56.39,12.1 56.05,12.45 56.05,15.7 63.45,23.11 v81.03,23.11
  Bottom 0.203: U9.1 81.09,23.05 v81.03,23.11 | v60.45,12.83 U8.3
N$8  (via drill 0.38)
  Top 0.203: v42.42,19.3 42.42,20.24 40.25,22.4 25.14,22.4 20.78,18.04 v20.78,17.7
  Bottom 0.203: U4.1 42.48,19.24 v42.42,19.3 | U1.11 20.57,17.49 v20.78,17.7
N$9  (via drill 0.38)
  Top 0.203: v79.63,20.19 77.77,22.05 63.9,22.05 60.45,18.6 v60.45,17.78 | v81.66,16.38 81.66,20.45 v81.03,21.08
  Bottom 0.203: v81.03,21.08 80.96,21.15 U9.4 79.73,20.29 v79.63,20.19 | v60.45,17.78 U8.12 | U10.1 81.66,16.09 v81.66,16.38
N$10  (via drill 0.38)
  Top 0.203: v81.03,19.3 81.03,20.24 78.86,22.4 63.75,22.4 59.39,18.04 v59.39,17.7
  Bottom 0.203: U11.1 81.09,19.24 v81.03,19.3 | U8.11 59.18,17.49 v59.39,17.7
N$11
  Bottom 0.457: R12.2 R11.1
N$12
  Bottom 0.457: Q2.3 66.76,14.05 66.93,14.22 R12.1
N$13  (via drill 0.38)
  Top 0.203: v42.42,82.3 41.76,82.96 24.99,82.96 18.03,76 v18.03,72.9
  Bottom 0.203: U16.2 v42.42,82.3 | v18.03,72.9 U15.6
N$14  (via drill 0.38)
  Top 0.203: v21.84,73.03 20.27,73.03 19.55,72.3 17.79,72.3 17.44,72.65 17.44,75.9 24.85,83.31 v42.42,83.31
  Bottom 0.203: U16.1 42.48,83.25 v42.42,83.31 | v21.84,73.03 U15.3
N$15  (via drill 0.38)
  Top 0.203: v41.02,80.39 39.17,82.25 25.29,82.25 21.84,78.8 v21.84,77.98 | v43.05,76.58 43.05,80.65 v42.42,81.28
  Bottom 0.203: v42.42,81.28 42.35,81.35 U16.4 41.12,80.49 v41.02,80.39 | v21.84,77.98 U15.12 | U17.1 43.05,76.29 v43.05,76.58
N$16  (via drill 0.38)
  Top 0.203: v42.42,79.5 42.42,80.44 40.25,82.6 25.14,82.6 20.78,78.24 v20.78,77.9
  Bottom 0.203: U18.1 42.48,79.44 v42.42,79.5 | U15.11 20.57,77.69 v20.78,77.9
N$17
  Bottom 0.457: R18.2 R17.1
N$18
  Bottom 0.457: Q3.3 28.15,74.25 28.32,74.42 R18.1
N$19  (via drill 0.38)
  Top 0.203: v81.03,82.3 80.37,82.96 63.6,82.96 56.64,76 v56.64,72.9
  Bottom 0.203: U23.2 v81.03,82.3 | v56.64,72.9 U22.6
N$20  (via drill 0.38)
  Top 0.203: v60.45,73.03 58.88,73.03 58.16,72.3 56.39,72.3 56.05,72.65 56.05,75.9 63.45,83.31 v81.03,83.31
  Bottom 0.203: U23.1 81.09,83.25 v81.03,83.31 | v60.45,73.03 U22.3
N$21  (via drill 0.38)
  Top 0.203: v79.63,80.39 77.77,82.25 63.9,82.25 60.45,78.8 v60.45,77.98 | v81.66,76.58 81.66,80.65 v81.03,81.28
  Bottom 0.203: v81.03,81.28 80.96,81.35 U23.4 79.73,80.49 v79.63,80.39 | v60.45,77.98 U22.12 | U24.1 81.66,76.29 v81.66,76.58
N$22  (via drill 0.38)
  Top 0.203: v81.03,79.5 81.03,80.44 78.86,82.6 63.75,82.6 59.39,78.24 v59.39,77.9
  Bottom 0.203: U25.1 81.09,79.44 v81.03,79.5 | U22.11 59.18,77.69 v59.39,77.9
N$23
  Bottom 0.457: R24.2 R23.1
N$24
  Bottom 0.457: Q4.3 66.76,74.25 66.93,74.42 R24.1
SCLK  (via drill 0.38)
  Top 0.203: v32.83,17.79 33.93,18.89 v33.93,20.07
  Bottom 0.203: U5.P$34 v33.93,20.07 | U6.1 29.7,16.55 31.19,18.04 32,18.04 32.24,17.79 v32.83,17.79
SCLK1  (via drill 0.38)
  Top 0.203: v71.44,17.79 72.54,18.89 v72.54,20.07
  Bottom 0.203: U14.P$34 v72.54,20.07 | U12.1 68.3,16.55 69.8,18.04 70.61,18.04 70.85,17.79 v71.44,17.79
SCLK2  (via drill 0.38)
  Top 0.203: v32.83,77.99 33.93,79.09 v33.93,80.26
  Bottom 0.203: U21.P$34 v33.93,80.26 | U19.1 29.7,76.74 31.19,78.23 32,78.23 32.24,77.99 v32.83,77.99
SCLK3  (via drill 0.38)
  Top 0.203: v71.44,77.99 72.54,79.09 v72.54,80.26
  Bottom 0.203: U28.P$34 v72.54,80.26 | U26.1 68.3,76.74 69.8,78.23 70.61,78.23 70.85,77.99 v71.44,77.99
SCLK_IN
  Bottom 0.203: U6.20 29.7,10.29 29.44,10.03 25.62,10.03 24.91,9.32 22.02,9.32 J1.3
SCLK_IN1
  Bottom 0.203: U12.20 68.3,10.29 68.05,10.03 64.23,10.03 63.52,9.32 60.63,9.32 J2.3
SCLK_IN2
  Bottom 0.203: U19.20 29.7,70.48 29.44,70.23 25.62,70.23 24.91,69.52 22.02,69.52 J3.3
SCLK_IN3
  Bottom 0.203: U26.20 68.3,70.48 68.05,70.23 64.23,70.23 63.52,69.52 60.63,69.52 J4.3
VIN  (via drill 0.38)
  Top 0.61: J1.2 18.29,8.89 21.42,12.03 39.71,12.03 v40.13,12.44
  Bottom 0.203: U6.16 31.3,11.86 31.5,12.06 33.4,12.06 34.12,12.79 R2.2
  Bottom 0.457: J1.2 17.62,8.13 16.3,9.45 14.99,9.45 12.86,11.58 11.02,11.58 10.54,12.06 10.54,13.02 | U7.3 10.54,14.92 | 10.54,14.92 10.54,13.02 | C1.1 11.09,16.17 10.54,15.62 10.54,14.92 | U7.1 10.54,13.02
  Bottom 0.61: R2.2 R1.2 R3.2 R4.2 39.78,12.79 v40.13,12.44 | C2.1 C1.1
VIN1  (via drill 0.38)
  Top 0.61: J2.2 56.9,8.89 60.03,12.03 78.32,12.03 v78.74,12.44
  Bottom 0.203: U12.16 69.9,11.86 70.1,12.06 72.01,12.06 72.73,12.79 R9.2
  Bottom 0.457: J2.2 56.22,8.13 54.9,9.45 53.6,9.45 51.46,11.58 49.63,11.58 49.15,12.06 49.15,13.02 | U13.3 49.15,14.92 | 49.15,14.92 49.15,13.02 | C6.1 49.7,16.17 49.15,15.62 49.15,14.92 | U13.1 49.15,13.02
  Bottom 0.61: R9.2 R7.2 R8.2 R10.2 78.39,12.79 v78.74,12.44 | C7.1 C6.1
VIN2  (via drill 0.38)
  Top 0.61: J3.2 18.29,69.09 21.42,72.23 39.71,72.23 v40.13,72.64
  Bottom 0.203: U19.16 31.3,72.06 31.5,72.26 33.4,72.26 34.12,72.99 R15.2
  Bottom 0.457: J3.2 17.62,68.33 16.3,69.65 14.99,69.65 12.86,71.78 11.02,71.78 10.54,72.26 10.54,73.22 | U20.3 10.54,75.12 | 10.54,75.12 10.54,73.22 | C11.1 11.09,76.37 10.54,75.82 10.54,75.12 | U20.1 10.54,73.22
  Bottom 0.61: R15.2 R13.2 R14.2 R16.2 39.78,72.99 v40.13,72.64 | C12.1 C11.1
VIN3  (via drill 0.38)
  Top 0.61: J4.2 56.9,69.09 60.03,72.23 78.32,72.23 v78.74,72.64
  Bottom 0.203: U26.16 69.9,72.06 70.1,72.26 72.01,72.26 72.73,72.99 R21.2
  Bottom 0.457: J4.2 56.22,68.33 54.9,69.65 53.6,69.65 51.46,71.78 49.63,71.78 49.15,72.26 49.15,73.22 | U27.3 49.15,75.12 | 49.15,75.12 49.15,73.22 | C16.1 49.7,76.37 49.15,75.82 49.15,75.12 | U27.1 49.15,73.22
  Bottom 0.61: R21.2 R19.2 R20.2 R22.2 78.39,72.99 v78.74,72.64 | C17.1 C16.1
WRD
  Bottom 0.203: U6.4 30.9,14.47 33.43,17 U5.P$33
WRD1
  Bottom 0.203: U12.4 69.5,14.47 72.04,17 U14.P$33
WRD2
  Bottom 0.203: U19.4 30.9,74.67 33.43,77.2 U21.P$33
WRD3
  Bottom 0.203: U26.4 69.5,74.67 72.04,77.2 U28.P$33
WRD_IN
  Bottom 0.203: J1.6 29.3,8.13 30.49,9.32 30.5,9.32 30.9,9.72 U6.17
WRD_IN1
  Bottom 0.203: J2.6 67.91,8.13 69.1,9.32 69.11,9.32 69.5,9.72 U12.17
WRD_IN2
  Bottom 0.203: J3.6 29.3,68.33 30.49,69.52 30.5,69.52 30.9,69.92 U19.17
WRD_IN3
  Bottom 0.203: J4.6 67.91,68.33 69.1,69.52 69.11,69.52 69.5,69.92 U26.17

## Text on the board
Top: X01 | X01 | X01 | X01
Dimension: Route Out | Route Out | Route Out | Route Out | Route Out | Route Out | Route Out | Route Out | Route Out | Route Out
tPlace: 1 | 18 | 1 | 18 | 1 | 18 | 1 | 18
Milling: v-score | v-score | v-score | v-score | v-score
